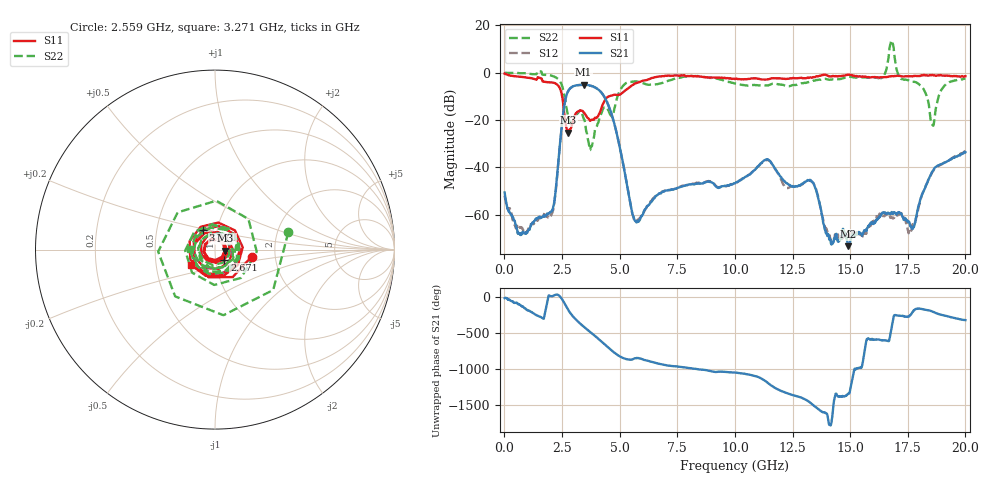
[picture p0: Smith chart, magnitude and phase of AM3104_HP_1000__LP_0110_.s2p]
!Created with skrf (http://scikit-rf.org).
# Hz S RI R 50.0
!freq ReS11 ImS11 ReS21 ImS21 ReS12 ImS12 ReS22 ImS22
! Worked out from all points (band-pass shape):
!   1601 points, 10 MHz to 20 GHz, reference 50 ohm
!   highest |S21| = -5.08 dB at 3.433 GHz (marker M1); lowest = -73.3 dB at 14.93 GHz (marker M2)
!   |S21| within 3 dB of the highest: 2.751 GHz to 4.185 GHz (1.434 GHz wide, 41.4 % of centre)
!   lowest |S11| = -25.3 dB at 2.771 GHz (marker M3), VSWR 1.12, Z = 55.7 - j0.717 ohm
!   |S11| at or under -10 dB: 2.506 GHz to 4.526 GHz (2.02 GHz wide, 57.4 % of centre)
!   |S22| runs from -32.7 to 13.6 dB; largest |S21 - S12| = 0.03
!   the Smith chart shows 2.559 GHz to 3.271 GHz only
!   S11 on the Smith chart (normalised r, x): 2.559 GHz: 1.51, -0.12; 2.671 GHz: 1.10, -0.12; 3.071 GHz: 0.86, +0.19; 3.271 GHz: 0.75, -0.13
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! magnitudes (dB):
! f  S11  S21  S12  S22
! 10 MHz  -0.4  -50.6  -52.0  0.0
! 672.2 MHz  -1.8  -68.4  -65.2  -0.2
! 2.009 GHz  -4.1  -58.9  -60.4  -1.2
! 2.559 GHz  -13.6  -16.7  -16.8  -7.5
! 2.671 GHz  -22.3  -10.3  -10.3  -13.4
! 2.771 GHz  -25.3  -7.7  -7.7  -18.9
! 3.071 GHz  -17.8  -5.5  -5.4  -18.1
! 3.271 GHz  -16.0  -5.1  -5.2  -17.0
! 3.346 GHz  -16.0  -5.1  -5.2  -16.9
! 3.433 GHz  -16.7  -5.1  -5.1  -19.3
! 3.746 GHz  -20.1  -5.5  -5.5  -31.5
! 4.545 GHz  -9.9  -14.6  -14.7  -16.8
! 5.657 GHz  -4.6  -62.4  -62.5  -3.7
! 6.682 GHz  -1.6  -51.4  -51.4  -4.8
! 10.01 GHz  -2.7  -46.8  -46.9  -4.6
! 13.34 GHz  -2.1  -46.0  -46.0  -3.6
! 14.18 GHz  -1.5  -72.2  -71.3  -3.0
! 14.93 GHz  -0.8  -73.3  -68.7  -1.7
! 16.68 GHz  -1.6  -59.5  -60.1  7.2
! 17.6 GHz  -1.5  -64.7  -67.0  -3.5
! 18.56 GHz  -0.9  -41.8  -42.0  -21.9
! 20 GHz  -1.5  -33.6  -33.2  -2.5
